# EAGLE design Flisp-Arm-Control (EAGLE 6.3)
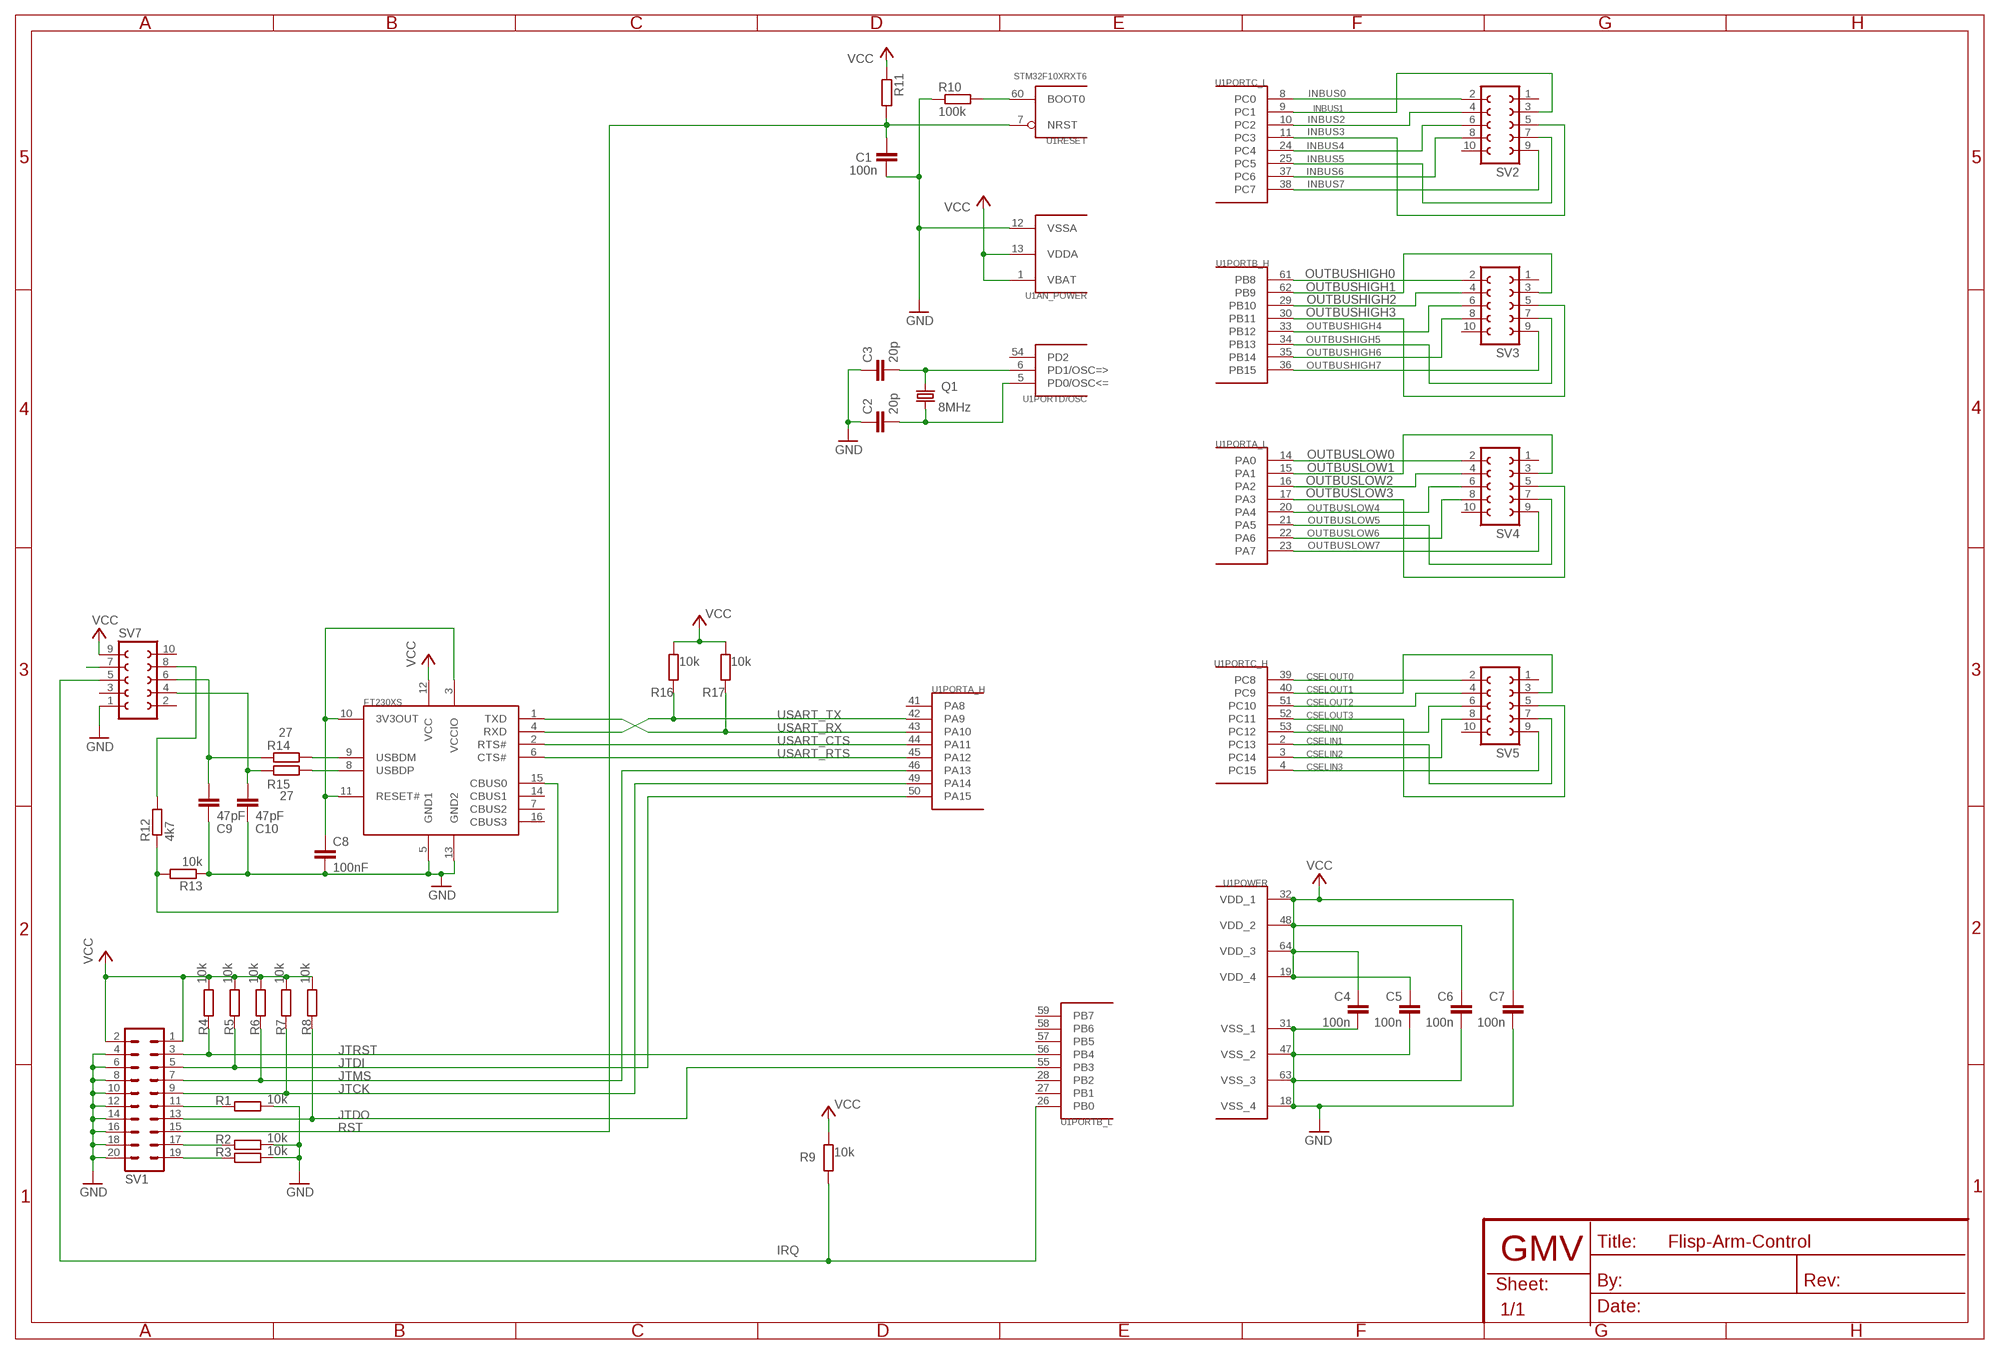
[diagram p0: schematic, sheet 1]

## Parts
C1  100n  C-EUC0603  [C0603]
C2  20p  C-EUC0603  [C0603]
C3  20p  C-EUC0603  [C0603]
C4  100n  C-EUC0603  [C0603]
C5  100n  C-EUC0603  [C0603]
C6  100n  C-EUC0603  [C0603]
C7  100n  C-EUC0603  [C0603]
C8  100nF  C-EUC0603  [C0603]
C9  47pF  C-EUC0603  [C0603]
C10  47pF  C-EUC0603  [C0603]
Q1  8MHz  CRYSTALSM49  [SM49]
R1  10k  R-EU_R0603  [R0603]
R2  10k  R-EU_R0603  [R0603]
R3  10k  R-EU_R0603  [R0603]
R4  10k  R-EU_R0603  [R0603]
R5  10k  R-EU_R0603  [R0603]
R6  10k  R-EU_R0603  [R0603]
R7  10k  R-EU_R0603  [R0603]
R8  10k  R-EU_R0603  [R0603]
R9  10k  R-EU_R0603  [R0603]
R10  100k  R-EU_R0603  [R0603]
R11  R-EU_R0603  [R0603]
R12  4k7  R-EU_R0603  [R0603]
R13  10k  R-EU_R0603  [R0603]
R14  27  R-EU_R0603  [R0603]
R15  27  R-EU_R0603  [R0603]
R16  10k  R-EU_R0603  [R0603]
R17  10k  R-EU_R0603  [R0603]
SV1  ML20  [ML20]
SV2  FE05-2  [FE05-2]
SV3  FE05-2  [FE05-2]
SV4  FE05-2  [FE05-2]
SV5  FE05-2  [FE05-2]
SV7  FE05-2  [FE05-2]
U1  STM32F10XRXT6  [TQFP64]
U2  FT230XS  [SSOP16-FTDI]

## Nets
CSELIN0: SV5.6 U1.53(PORTC_H:PC12)
CSELIN1: SV5.7 U1.2(PORTC_H:PC13)
CSELIN2: SV5.8 U1.3(PORTC_H:PC14)
CSELIN3: SV5.9 U1.4(PORTC_H:PC15)
CSELOUT0: SV5.2 U1.39(PORTC_H:PC8)
CSELOUT1: SV5.3 U1.40(PORTC_H:PC9)
CSELOUT2: SV5.4 U1.51(PORTC_H:PC10)
CSELOUT3: SV5.5 U1.52(PORTC_H:PC11)
GND: C1.1 C2.1 C3.1 C4.2 C5.2 C6.2 C7.2 C8.2 C9.2 C10.2 R1.2 R2.2 R3.2 R10.1 R13.1 SV1.4 SV1.6 SV1.8 SV1.10 SV1.12 SV1.14 SV1.16 SV1.18 SV1.20 SV7.1 U1.12(AN_POWER:VSSA) U1.18(POWER:VSS_4) U1.31(POWER:VSS_1) U1.47(POWER:VSS_2) U1.63(POWER:VSS_3) U2.5(GND1) U2.13(GND2)
INBUS0: SV2.2 U1.8(PORTC_L:PC0)
INBUS1: SV2.3 U1.9(PORTC_L:PC1)
INBUS2: SV2.4 U1.10(PORTC_L:PC2)
INBUS3: SV2.5 U1.11(PORTC_L:PC3)
INBUS4: SV2.6 U1.24(PORTC_L:PC4)
INBUS5: SV2.7 U1.25(PORTC_L:PC5)
INBUS6: SV2.8 U1.37(PORTC_L:PC6)
INBUS7: SV2.9 U1.38(PORTC_L:PC7)
IRQ: R9.1 SV7.5 U1.26(PORTB_L:PB0)
JTCK: R7.1 SV1.9 U1.49(PORTA_H:PA14)
JTDI: R5.1 SV1.5 U1.50(PORTA_H:PA15)
JTDO: R8.1 SV1.13 U1.55(PORTB_L:PB3)
JTMS: R6.1 SV1.7 U1.46(PORTA_H:PA13)
JTRST: R4.1 SV1.3 U1.56(PORTB_L:PB4)
N$2: R10.2 U1.60(RESET:BOOT0)
N$3: R12.2 SV7.8
N$4: SV7.7
N$319: R14.2 U2.9(USBDM)
N$321: R15.2 U2.8(USBDP)
N$322: C3.2 Q1.2 U1.6(PORTD/OSC:PD1/OSC=>)
N$323: C2.2 Q1.1 U1.5(PORTD/OSC:PD0/OSC<=)
N$325: R3.1 SV1.19
N$334: R2.1 SV1.17
N$336: R1.1 SV1.11
N$337: C8.1 U2.3(VCCIO) U2.10(3V3OUT) U2.11(RESET#)
N$352: R12.1 R13.2 U2.15(CBUS0)
N$354: C9.1 R14.1 SV7.6
N$355: C10.1 R15.1 SV7.4
OUTBUSHIGH0: SV3.2 U1.61(PORTB_H:PB8)
OUTBUSHIGH1: SV3.3 U1.62(PORTB_H:PB9)
OUTBUSHIGH2: SV3.4 U1.29(PORTB_H:PB10)
OUTBUSHIGH3: SV3.5 U1.30(PORTB_H:PB11)
OUTBUSHIGH4: SV3.6 U1.33(PORTB_H:PB12)
OUTBUSHIGH5: SV3.7 U1.34(PORTB_H:PB13)
OUTBUSHIGH6: SV3.8 U1.35(PORTB_H:PB14)
OUTBUSHIGH7: SV3.9 U1.36(PORTB_H:PB15)
OUTBUSLOW0: SV4.2 U1.14(PORTA_L:PA0)
OUTBUSLOW1: SV4.3 U1.15(PORTA_L:PA1)
OUTBUSLOW2: SV4.4 U1.16(PORTA_L:PA2)
OUTBUSLOW3: SV4.5 U1.17(PORTA_L:PA3)
OUTBUSLOW4: SV4.6 U1.20(PORTA_L:PA4)
OUTBUSLOW5: SV4.7 U1.21(PORTA_L:PA5)
OUTBUSLOW6: SV4.8 U1.22(PORTA_L:PA6)
OUTBUSLOW7: SV4.9 U1.23(PORTA_L:PA7)
RST: C1.2 R11.2 SV1.15 U1.7(RESET:NRST)
USART_CTS: U1.44(PORTA_H:PA11) U2.2(RTS#)
USART_RTS: U1.45(PORTA_H:PA12) U2.6(CTS#)
USART_RX: R17.1 U1.43(PORTA_H:PA10) U2.1(TXD)
USART_TX: R16.1 U1.42(PORTA_H:PA9) U2.4(RXD)
VCC: C4.1 C5.1 C6.1 C7.1 R4.2 R5.2 R6.2 R7.2 R8.2 R9.2 R11.1 R16.2 R17.2 SV1.1 SV1.2 SV7.9 U1.1(AN_POWER:VBAT) U1.13(AN_POWER:VDDA) U1.19(POWER:VDD_4) U1.32(POWER:VDD_1) U1.48(POWER:VDD_2) U1.64(POWER:VDD_3) U2.12(VCC)
Unconnected: SV2.1 SV2.10 SV3.1 SV3.10 SV4.1 SV4.10 SV5.1 SV5.10 SV7.2 SV7.3 SV7.10 U1.27(PORTB_L:PB1) U1.28(PORTB_L:PB2) U1.41(PORTA_H:PA8) U1.54(PORTD/OSC:PD2) U1.57(PORTB_L:PB5) U1.58(PORTB_L:PB6) U1.59(PORTB_L:PB7) U2.7(CBUS2) U2.14(CBUS1) U2.16(CBUS3)

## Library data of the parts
C1-C10 = rcl:C-EU: CAPACITOR, European symbol
Q1 = crystal:CRYSTAL: CRYSTAL; OC_FARNELL: unknown; OC_NEWARK: unknown
R1-R17 = rcl:R-EU_: RESISTOR, European symbol
SV1 = con-harting-ml:ML20: HARTING; OC_FARNELL: unknown; OC_NEWARK: unknown
SV2-SV5 SV7 = con-lsta:FE05-2: FEMALE HEADER; OC_FARNELL: unknown; OC_NEWARK: unknown
U1 = stm32:STM32F10XRXT6: STM32F101/103 64pin LQFP
U2 = 0misc:FT230X

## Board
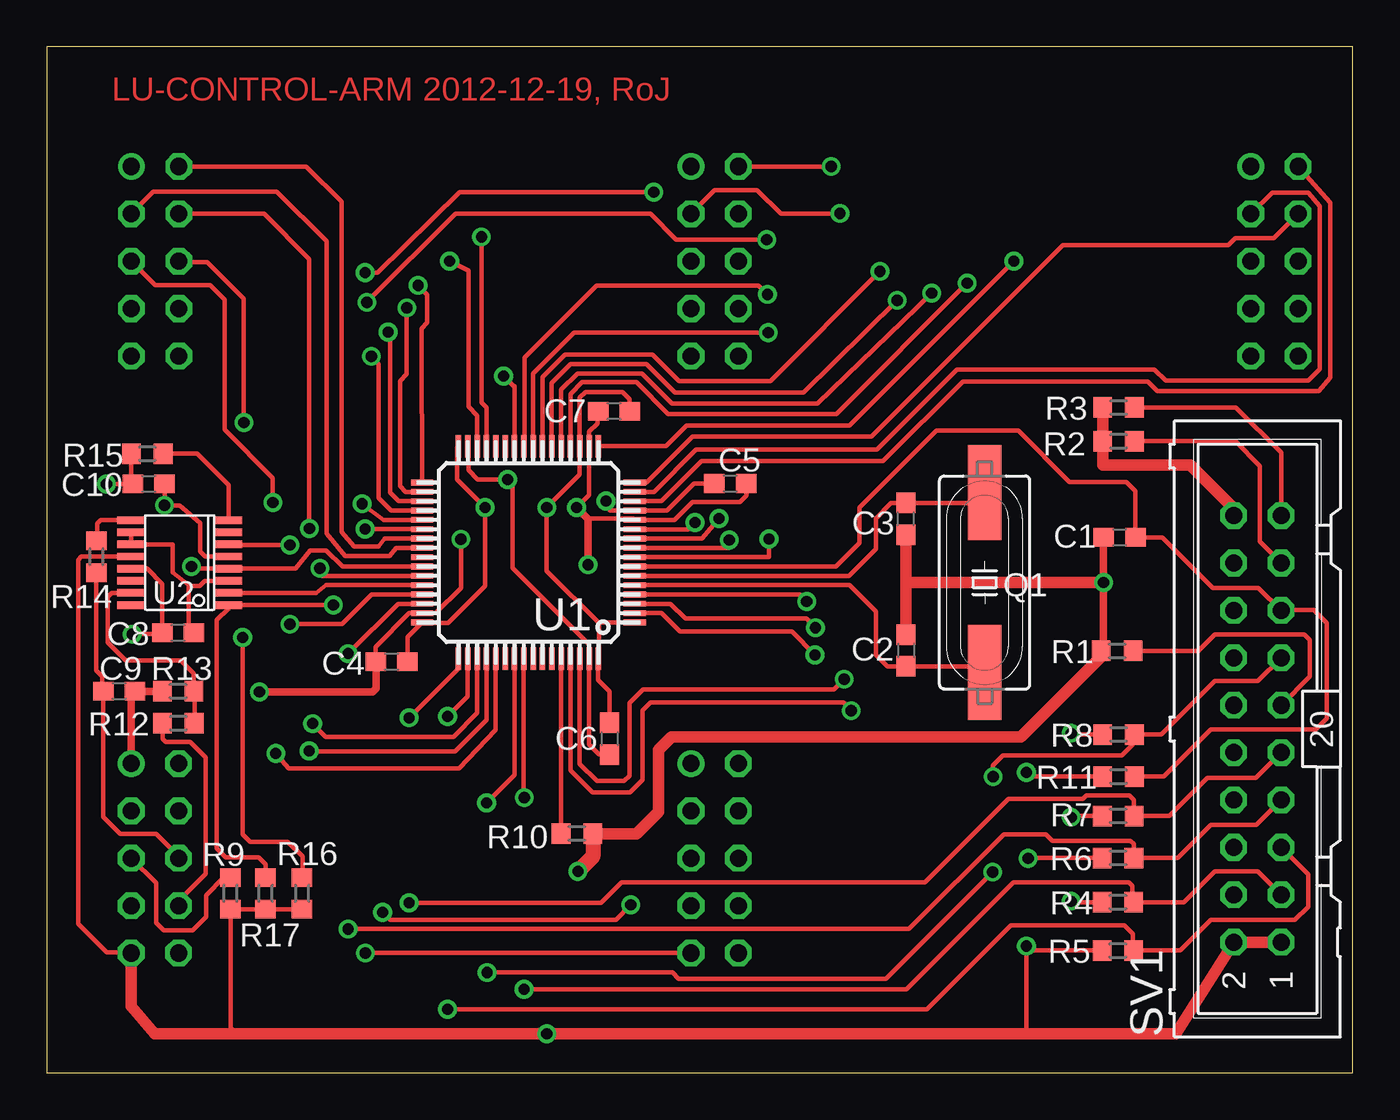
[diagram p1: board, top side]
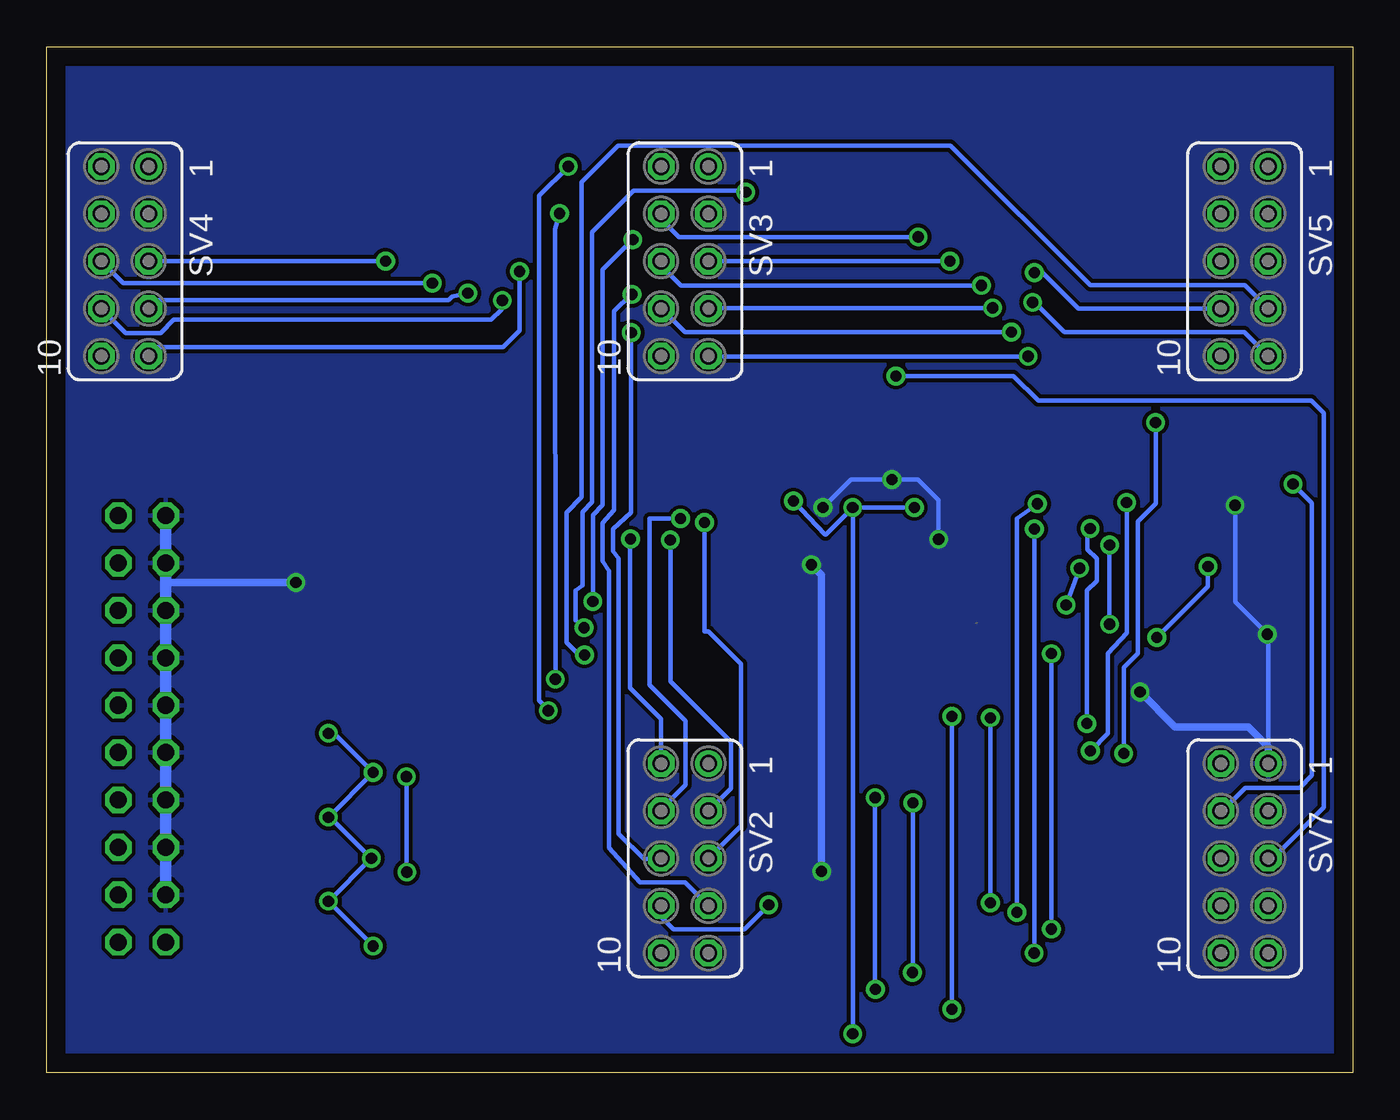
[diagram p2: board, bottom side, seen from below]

Size 70 x 55 mm. Coordinates in mm from the lower left corner, seen from the top.
Outline: 0,0 70,0 70,55 0,55 0,0
Copper layers (1*16): Top 0.035mm / dielectric 1.5mm / Bottom 0.035mm
Design rules "default *": minimum track width 10mil, minimum drill 12mil, track to track 8mil, track to pad 8mil, pad to pad 8mil, via to via 8mil, smd to smd 0mil, copper to edge 40mil, drill to drill 8mil, minimum pad ring 10mil, minimum via ring 8mil, stop-mask expansion 4mil, vias tented up to drill 0mil, thermal gap 10mil

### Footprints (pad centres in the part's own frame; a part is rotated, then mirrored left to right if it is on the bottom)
C0603 = smd 1.1 x 1: 1 -0.85,0; 2 0.85,0
SM49 = smd 5.08 x 1.778: 1 -4.826,0; 2 4.826,0
R0603 = smd 1 x 1.1: 1 -0.85,0; 2 0.85,0
ML20 = drill 0.914 octagon: 1 -11.43,-1.27; 2 -11.43,1.27; 3 -8.89,-1.27; 4 -8.89,1.27; 5 -6.35,-1.27; 6 -6.35,1.27; 7 -3.81,-1.27; 8 -3.81,1.27; 9 -1.27,-1.27; 10 -1.27,1.27; 11 1.27,-1.27; 12 1.27,1.27; 13 3.81,-1.27; 14 3.81,1.27; 15 6.35,-1.27; 16 6.35,1.27; 17 8.89,-1.27; 18 8.89,1.27; 19 11.43,-1.27; 20 11.43,1.27
FE05-2 = drill 0.914: 1 -5.08,1.27 | drill 0.914 octagon: 2 -5.08,-1.27; 3 -2.54,1.27; 4 -2.54,-1.27; 5 0,1.27; 6 0,-1.27; 7 2.54,1.27; 8 2.54,-1.27; 9 5.08,1.27; 10 5.08,-1.27
TQFP64 = smd 1.2 x 0.3: 1 -5.7,3.75; 2 -5.7,3.25; 3 -5.7,2.75; 4 -5.7,2.25; 5 -5.7,1.75; 6 -5.7,1.25; 7 -5.7,0.75; 8 -5.7,0.25; 9 -5.7,-0.25; 10 -5.7,-0.75; 11 -5.7,-1.25; 12 -5.7,-1.75; 13 -5.7,-2.25; 14 -5.7,-2.75; 15 -5.7,-3.25; 16 -5.7,-3.75; 33 5.7,-3.75; 34 5.7,-3.25; 35 5.7,-2.75; 36 5.7,-2.25; 37 5.7,-1.75; 38 5.7,-1.25; 39 5.7,-0.75; 40 5.7,-0.25; 41 5.7,0.25; 42 5.7,0.75; 43 5.7,1.25; 44 5.7,1.75; 45 5.7,2.25; 46 5.7,2.75; 47 5.7,3.25; 48 5.7,3.75 | smd 0.3 x 1.2: 17 -3.75,-5.7; 18 -3.25,-5.7; 19 -2.75,-5.7; 20 -2.25,-5.7; 21 -1.75,-5.7; 22 -1.25,-5.7; 23 -0.75,-5.7; 24 -0.25,-5.7; 25 0.25,-5.7; 26 0.75,-5.7; 27 1.25,-5.7; 28 1.75,-5.7; 29 2.25,-5.7; 30 2.75,-5.7; 31 3.25,-5.7; 32 3.75,-5.7; 49 3.75,5.7; 50 3.25,5.7; 51 2.75,5.7; 52 2.25,5.7; 53 1.75,5.7; 54 1.25,5.7; 55 0.75,5.7; 56 0.25,5.7; 57 -0.25,5.7; 58 -0.75,5.7; 59 -1.25,5.7; 60 -1.75,5.7; 61 -2.25,5.7; 62 -2.75,5.7; 63 -3.25,5.7; 64 -3.75,5.7
SSOP16-FTDI = smd 0.4 x 1.5: 1 -2.275,-2.609; 2 -1.625,-2.609; 3 -0.975,-2.609; 4 -0.325,-2.609; 5 0.325,-2.609; 6 0.975,-2.609; 7 1.625,-2.609; 8 2.275,-2.609; 9 2.275,2.609; 10 1.625,2.609; 11 0.975,2.609; 12 0.325,2.609; 13 -0.325,2.609; 14 -0.975,2.609; 15 -1.625,2.609; 16 -2.275,2.609

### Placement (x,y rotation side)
C1  57.5,28.7 0 top
C2  46.05,22.64 270 top
C3  46.05,29.7 90 top
C4  18.49,22.03 180 top
C5  36.63,31.58 0 top
C6  30.17,17.91 270 top
C7  30.4,35.46 180 top
C8  7.05,23.58 180 top
C9  3.89,20.46 0 top
C10  5.47,31.57 0 top
Q1  50.27,26.28 90 top
R1  57.37,22.62 180 top
R2  57.44,33.85 180 top
R3  57.44,35.66 180 top
R4  57.41,9.15 180 top
R5  57.4,6.55 180 top
R6  57.41,11.52 180 top
R7  57.43,13.77 180 top
R8  57.44,18.14 180 top
R9  9.85,9.62 270 top
R10  28.42,12.83 180 top
R11  57.44,15.88 0 top
R12  7.06,18.74 180 top
R13  7.05,20.45 0 top
R14  2.67,27.66 90 top
R15  5.39,33.18 0 top
R16  13.69,9.62 270 top
R17  11.73,9.62 270 top
SV1  64.89,18.43 90 top
SV2  35.8,11.5 270 bottom
SV3  35.8,43.5 270 bottom
SV4  65.8,43.5 270 bottom
SV5  5.81,43.5 270 bottom
SV7  5.8,11.5 270 bottom
U1  25.82,27.89 180 top
U2  7.13,27.35 90 top

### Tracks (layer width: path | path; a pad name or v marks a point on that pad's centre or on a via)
CSELIN0  (via drill 0.6)
  Top 0.254: U1.53 24.07,18.38 22.11,16.32 12.98,16.32 v12.28,17.12 | v10.57,34.85 10.57,41.49 8.6,43.46 7.12,43.46 SV5.6
  Bottom 0.254: v12.28,17.12 12.28,21.72 11.53,22.47 11.53,29.56 10.57,30.52 v10.57,34.85
CSELIN1  (via drill 0.6)
  Top 0.254: U1.2 32.94,24.64 33.93,23.65 39.93,23.65 v41.18,22.4
  Bottom 0.254: v41.18,22.4 41.46,22.4 42.14,23.08 42.14,30.04 41.33,30.85 41.33,47.75 39.39,49.69 21.56,49.69 14.08,42.21 5.79,42.21 SV5.7
CSELIN2  (via drill 0.6)
  Top 0.254: U1.3 33.43,25.14 34.23,24.34 40.72,24.34 v41.2,23.86 | v32.54,47.2 22.12,47.2 17.74,42.9 v17.08,42.9 v17.07,42.89
  Bottom 0.254: v41.2,23.86 41.2,23.89 41.66,24.25 41.66,25.86 41.29,26.13 41.29,30.07 40.77,30.59 40.77,45.05 38.55,47.27 32.61,47.27 v32.54,47.2 | v17.07,42.89 16.65,42.89 14.71,40.95 SV5.8
CSELIN3  (via drill 0.6)
  Top 0.254: U1.4 40.36,25.64 v40.73,25.27 | v38.59,44.66 33.74,44.66 32.35,46.05 21.91,46.05 v17.16,41.3
  Bottom 0.254: v40.73,25.27 40.73,29.91 40.2,30.44 40.2,43.05 v38.59,44.66 | v17.16,41.3 17.07,41.3 15.46,39.69 5.81,39.69 SV5.9
CSELOUT0
  Top 0.254: U1.39 18.1,28.64 17.78,28.22 16.48,28.22 15.8,29 15.8,46.69 13.91,48.58 SV5.2
CSELOUT1
  Top 0.254: U1.40 18.72,28.14 18.38,27.7 16,27.7 15,28.9 15,44.57 12.33,47.24 5.72,47.24 4.54,46.06 SV5.3
CSELOUT2  (via drill 0.6)
  Top 0.254: U1.51 23.07,19.28 21.8,18.01 14.96,18.01 v14.25,18.72 | v14.08,29.18 14.08,43.62 11.66,46.04 SV5.4
  Bottom 0.254: v14.25,18.72 14.25,25.85 13.73,26.37 13.73,27.56 14.23,28.06 14.23,29.03 v14.08,29.18
CSELOUT3  (via drill 0.6)
  Top 0.254: U1.52 23.57,18.91 21.9,17.24 v14.07,17.24 v14.06,17.25 | v12.12,30.56 12.12,31.89 9.53,34.48 9.53,41.44 8.75,42.22 5.82,42.22 SV5.5
  Bottom 0.254: v14.06,17.25 v14.05,17.25 13.12,18.18 13.12,22.47 12.12,23.57 v12.12,30.56
GND  (via drill 0.6)
  Top 0.254: C6.2 29.6,17.06 29.06,17.6 U1.63 29.07,22.95 24.97,27.05 24.97,31.53 v24.7,31.8 23.1,31.8 22.6,32.3 22.6,33.56 U1.31 | C4.2 17.62,22.05 17.62,22.83 19.43,24.64 U1.47 20.84,24.64 22.2,26 v22.2,28.6 | C7.2 29.51,35.42 29.51,34.81 29.07,34.37 U1.18 29.07,30.97 v28.4,30.3 29,29.7 31.46,29.7 U1.12 33.64,29.64 34.6,30.6 37.15,30.6 37.5,30.95 37.5,31.56 C5.2 | U2.13 5.38,27.02 6.2,26.2 C8.2 6.13,23.51 v4.59,23.51 | 4.53,20.25 C9.2 R13.1 | C10.2 v6.32,30.43 v6.31,30.42 6.33,30.4 7.12,30.4 8.24,29.48 8.24,27.94 8.51,27.68 U2.5
  Top 0.406: C1.1 56.61,28.74 56.58,28.74 56.64,28.68 v56.64,26.28 56.64,22.74 R1.2 | v29.01,27.23 29.01,29.69 v28.4,30.3 | v11.4,20.42 17.46,20.42 17.65,20.61 C4.2 | R13.1 4.53,20.45 SV7.1
  Top 0.61: C2.1 C3.1 46.05,26.28 v56.64,26.28 | R3.2 R2.2 56.59,32.57 61.3,32.57 63.62,30.25 SV1.20 | 56.64,22.74 56.64,22.43 52.22,18.01 33.48,18.01 32.79,17.32 32.79,14 31.61,12.82 R10.1
  Top 0.813: R10.1 29.27,11.6 v28.47,10.8
  Bottom 0.254: v22.2,28.6 22.2,30.7 23.3,31.8 v24.7,31.8 26.9,31.8 v28.4,30.3 | v6.31,30.42 6.31,25.23 v4.59,23.51 4.53,23.45 SV7.1
  Bottom 0.406: v56.64,26.28 63.62,26.28 | v28.47,10.8 28.47,26.69 v29.01,27.23 | SV7.1 4.53,17.48 5.6,18.55 9.53,18.55 v11.4,20.42
  Bottom 0.61: SV1.4 SV1.6 SV1.8 SV1.10 SV1.12 SV1.14 SV1.16 63.62,26.28 SV1.18 SV1.20
  pour Bottom: 0,55 70,55 70,0 0,0
INBUS0  (via drill 0.6)
  Top 0.254: U1.8 38.71,27.65 v38.71,28.61
  Bottom 0.254: SV2.2 37.07,18.96 38.74,20.63 38.74,28.58 v38.71,28.61
INBUS1  (via drill 0.6)
  Top 0.254: U1.9 36.38,28.14 36.58,28.13 v36.58,28.56
  Bottom 0.254: v36.58,28.56 36.58,20.99 33.32,17.73 33.32,15.25 SV2.3
INBUS2  (via drill 0.6)
  Top 0.254: v36.03,29.71 35.12,28.64 U1.10
  Bottom 0.254: v36.03,29.71 37.69,29.71 37.69,20.79 35.77,18.87 35.77,15.42 37.07,14.12 SV2.4
INBUS3  (via drill 0.6)
  Top 0.254: U1.11 34.38,29.13 v34.75,29.5
  Bottom 0.254: v34.75,29.5 34.74,23.66 34.53,23.66 32.78,21.91 32.78,13.25 SV2.5
INBUS4  (via drill 0.6)
  Top 0.254: 26.1,33.62 U1.24 26.07,37.48 28.27,39.68 v38.66,39.68 v38.67,39.67
  Bottom 0.254: v38.67,39.67 38.67,30.03 39.65,29.15 39.65,27.97 39.36,27.58 39.36,12.82 38,11.46 37.11,11.46 SV2.6
INBUS5  (via drill 0.6)
  Top 0.254: U1.25 25.6,33.62 25.6,38.34 29.46,42.2 38.15,42.2 v38.63,41.72
  Bottom 0.254: v38.63,41.72 38.69,41.72 39.59,40.82 39.59,30.17 40.2,29.46 40.2,27.44 39.86,26.9 39.86,12.07 38.21,10.22 35.79,10.22 SV2.7
INBUS6  (via drill 0.6)
  Top 0.254: U1.37 18.06,29.64 v16.9,30.5 | v18,8.6 18.4,8.2 30.5,8.2 v31.3,9
  Bottom 0.254: v16.9,30.5 18,29.7 v18,8.6 | v31.3,9 32.6,7.7 36.4,7.7 37.07,8.37 SV2.8
INBUS7  (via drill 0.6)
  Top 0.254: U1.38 v17.06,29.14 | v17.08,6.42 SV2.9
  Bottom 0.254: v17.06,29.14 17.07,20.82 v17.07,6.43 v17.08,6.42
IRQ  (via drill 0.6)
  Top 0.254: U1.26 25.07,36.81 25.03,36.81 v24.49,37.35 | R9.1 9.49,10.47 8.54,9.52 8.54,8.36 7.82,7.64 6.26,7.64 5.86,8.04 5.86,10.17 SV7.5
  Bottom 0.254: v24.49,37.35 18.18,37.35 16.86,36.03 2.22,36.03 1.56,35.37 1.56,14.24 4.3,11.5 SV7.5
JTCK  (via drill 0.6)
  Top 0.254: SV1.9 64.79,15.8 62.2,15.8 60.17,13.77 R7.1 58.26,13.79 58.26,14.62 58.02,14.86 55.72,14.86 55.53,14.67 51.53,14.67 47.08,10.22 33.72,10.22 30.81,10.21 29.7,9.1 v19.43,9.11 | U1.49 22.07,21.67 v19.43,19.03
  Bottom 0.254: v19.43,19.03 v19.43,9.11
JTDI  (via drill 0.6)
  Top 0.254: SV1.5 67.6,10.64 67.6,8.9 66.9,8.2 62.4,8.2 60.76,6.55 R5.1 58.22,6.59 58.22,7.45 57.76,7.91 51.68,7.91 47.18,3.41 v21.49,3.41 | U1.50 22.57,20.18 v21.49,19.1
  Bottom 0.254: v21.49,19.1 v21.49,3.41
JTDO  (via drill 0.6)
  Top 0.254: SV1.13 64.91,21 62.6,21 59.74,18.14 R8.1 58.22,18.21 58.22,17.6 57.63,17.01 51.24,17.01 50.72,16.49 v50.72,15.88 | U1.55 25.07,15.96 v23.58,14.47 | v23.61,5.38 33.53,5.38 33.86,5.05 44.99,5.05 v50.7,10.76
  Bottom 0.254: v23.58,14.47 23.58,5.41 v23.61,5.38 | v50.7,10.76 50.7,15.86 v50.72,15.88
JTMS  (via drill 0.6)
  Top 0.254: SV1.7 64.83,13.3 62.4,13.3 60.62,11.52 R6.1 58.25,12.27 58.08,12.44 53.9,12.44 53.56,12.78 51.29,12.78 46.22,7.71 v16.15,7.71 | U1.46 18.83,25.14 v16.16,22.47
  Bottom 0.254: v16.16,22.47 v16.16,7.72 v16.15,7.71
JTRST  (via drill 0.6)
  Top 0.254: SV1.3 64.9,10.8 62.6,10.8 60.95,9.15 R4.1 58.19,9.21 58.19,10.01 57.99,10.21 51.8,10.21 46.07,4.48 v25.58,4.48 | U1.56 25.57,14.78 v25.6,14.75
  Bottom 0.254: v25.6,14.75 25.6,4.5 v25.58,4.48
N$2
  Top 0.254: U1.60 R10.2
N$3
  Top 0.254: SV7.8 7.07,9.22 8.51,10.66 8.51,16.91 7.69,17.73 6.39,17.73 6.21,17.91 R12.2
N$319
  Top 0.254: U2.9 2.9,29.62 2.7,29.43 2.7,28.61 R14.2
N$321
  Top 0.254: R15.2 8.08,33.18 9.75,31.51 9.75,29.64 U2.8
N$322
  Top 0.254: U1.6 43,26.64 44.44,28.08 44.44,29.72 45.25,30.53 46.03,30.53 C3.2 49.71,30.55 | Q1.2 49.83,30.67 49.71,30.55 | 49.71,30.55 49.5,30.34
N$323
  Top 0.254: U1.5 43.02,26.14 44.44,24.72 44.44,22.41 45.07,21.78 C2.2 49.93,21.79 Q1.1
N$325
  Top 0.254: R3.1 63.74,35.66 66.16,33.24 SV1.19
N$334
  Top 0.254: R2.1 63.69,33.85 65.01,32.53 65.01,28.47 SV1.17
N$336
  Top 0.254: R1.1 61.72,22.62 62.6,23.5 67.4,23.5 67.7,23.2 67.7,21.25 SV1.11
N$337
  Top 0.254: U2.10 U2.11 4.54,28.31 6.76,28.31 6.76,26.83 7.61,26.16 7.6,26.18 | C8.1 7.6,23.88 7.6,26.18 | U2.3 8.47,26.38 8.2,26.1 7.67,26.1 7.6,26.18
N$352
  Top 0.254: R12.1 7.91,18.8 7.92,18.81 7.92,20.43 R13.2 7.88,20.47 7.88,21.41 7.19,22.1 4.23,22.1 3.26,23.07 3.26,25.5 3.48,25.73 U2.15
N$354
  Top 0.254: SV7.6 7.07,11.59 5.86,12.8 3.95,12.8 3.03,13.72 C9.1 2.99,20.51 2.99,21.24 2.67,21.56 R14.1
N$355  (via drill 0.6)
  Top 0.254: v3.21,31.56 C10.1 4.54,31.64 R15.1
  Bottom 0.254: SV7.4 7.01,14.04 5.77,15.28 2.85,15.28 2.2,15.93 2.2,30.55 v3.21,31.56
OUTBUSHIGH0  (via drill 0.6)
  Top 0.254: U1.61 28.07,16.2 29.25,15.02 31.26,15.02 31.94,15.7 31.94,19.43 32.35,19.84 42.69,19.84 v43.12,19.41 | v42.04,48.58 SV3.2
  Bottom 0.254: v43.12,19.41 43.12,19.47 43.61,19.96 43.61,47.01 v42.04,48.58
OUTBUSHIGH1  (via drill 0.6)
  Top 0.254: U1.62 28.57,16.56 29.49,15.64 30.95,15.64 31.23,15.92 31.23,19.82 31.96,20.55 42.19,20.55 v42.74,21.1 | v42.51,46.06 39.34,46.04 38.08,47.3 35.79,47.3 SV3.3
  Bottom 0.254: v42.74,21.1 42.76,45.21 v42.51,46.06
OUTBUSHIGH2  (via drill 0.6)
  Top 0.254: U1.29 23.57,35.65 23.3,35.92 v23.3,44.8
  Bottom 0.254: SV3.4 37.07,45.77 36.1,44.8 v23.3,44.8
OUTBUSHIGH3  (via drill 0.6)
  Top 0.254: U1.30 23.07,35.24 22.6,35.71 22.6,43 v21.59,43.51
  Bottom 0.254: v21.59,43.51 SV3.5
OUTBUSHIGH4  (via drill 0.6)
  Top 0.254: v19.9,42.2 20.4,41.7 20.4,40.2 20.1,39.9 20.1,39 U1.33
  Bottom 0.254: SV3.6 37.17,43.4 37.2,43.4 36,42.2 v19.9,42.2
OUTBUSHIGH5  (via drill 0.6)
  Top 0.254: U1.34 19.24,31.14 18.93,31.45 18.93,37.08 19.3,37.45 v19.3,41
  Bottom 0.254: SV3.7 34.49,41 21.1,41 21,41 v19.3,41
OUTBUSHIGH6  (via drill 0.6)
  Top 0.254: U1.35 18.86,30.64 18.4,31.1 18.4,39.6 v18.3,39.7
  Bottom 0.254: SV3.8 37.1,40.99 37.1,41 35.8,39.7 20.8,39.7 20.5,39.7 v18.3,39.7
OUTBUSHIGH7  (via drill 0.6)
  Top 0.254: U1.36 18.46,30.14 17.8,30.8 17.8,38 v17.4,38.4
  Bottom 0.254: SV3.9 34.51,38.4 v17.4,38.4
OUTBUSLOW0
  Top 0.254: U1.14 32.94,30.64 35.1,32.8 44.83,32.8 49.09,37.06 59,37.06 59.52,36.54 68.17,36.54 68.8,37.27 68.8,46.65 SV4.2
OUTBUSLOW1
  Top 0.254: U1.15 32.54,31.14 34.8,33.4 44.5,33.4 48.79,37.69 59.37,37.69 59.97,37.09 67.61,37.09 68.24,37.72 68.24,46.46 67.62,47.18 65.67,47.18 SV4.3
OUTBUSLOW2
  Top 0.254: U1.16 32.14,31.64 34.6,34.1 44.2,34.1 54.47,44.37 63.33,44.37 63.69,44.73 65.76,44.73 SV4.4
OUTBUSLOW3  (via drill 0.6)
  Top 0.254: U1.17 33.19,33.59 34.29,34.69 43.03,34.69 v51.84,43.5
  Bottom 0.254: v51.84,43.5 SV4.5
OUTBUSLOW4  (via drill 0.6)
  Top 0.254: U1.20 28.07,36.39 28.69,37.01 31.62,37.01 33.31,35.32 36.77,35.32 | 36.77,35.32 36.78,35.31 | 36.77,35.32 42.33,35.32 v49.33,42.32
  Bottom 0.254: v49.33,42.32 65.89,42.32 SV4.6
OUTBUSLOW5  (via drill 0.6)
  Top 0.254: U1.21 27.57,36.61 28.44,37.48 31.9,37.48 33.52,35.86 41.3,35.86 v47.43,41.79
  Bottom 0.254: v47.43,41.79 48.28,41.59 48.46,41.41 64.08,41.41 SV4.7
OUTBUSLOW6  (via drill 0.6)
  Top 0.254: U1.22 27.07,36.97 28.08,37.98 32.15,37.98 33.67,36.46 36.73,36.46 36.74,36.47 40.55,36.47 v45.58,41.4
  Bottom 0.254: v45.58,41.4 45.63,40.9 46.17,40.36 63.18,40.36 63.88,39.66 65.77,39.66 SV4.8
OUTBUSLOW7  (via drill 0.6)
  Top 0.254: U1.23 26.57,37.29 27.78,38.5 32.46,38.5 33.88,37.08 38.78,37.08 v44.66,42.96
  Bottom 0.254: v44.66,42.96 44.66,39.79 45.54,38.91 64.04,38.91 SV4.9
RST
  Top 0.254: U1.7 42.31,27.14 43.56,28.39 43.56,30.3 47.68,34.42 52.07,34.42 54.82,31.67 57.87,31.67 58.35,31.19 C1.2 | 58.28,28.77 C1.2 | R11.2 59.88,15.88 62.4,18.4 68,18.4 68.6,19 68.6,24.1 67.9,24.8 66.17,24.8 SV1.15 64.94,26 62.5,26 59.8,28.7 C1.2
USART_CTS
  Top 0.254: U1.44 14.97,26.15 14.45,25.73 U2.2
USART_RTS  (via drill 0.6)
  Top 0.254: U2.6 9.77,28.29 v13.04,28.29 | v13.04,24.05 14.8,24.05 14.78,24.05 15.84,24.05 17.42,25.64 U1.45
  Bottom 0.254: v13.04,28.29 v13.04,24.05
USART_RX  (via drill 0.6)
  Top 0.254: U2.1 | U2.1 v15.37,25.07 | v14.64,27.05 14.75,26.64 U1.43 | U2.1 9.74,24.89 9.11,24.26 9.11,12.03 9.59,11.55 11.35,11.55 11.73,11.17 R17.1
  Bottom 0.254: v15.37,25.07 15.34,25.1 v14.64,27.05
USART_TX  (via drill 0.6)
  Top 0.254: U1.42 15.85,27.14 14.99,28 14.11,28 13.35,27.04 9.75,27.04 U2.4 7.88,27.02 v7.76,27.14 | v10.51,23.33 10.51,12.78 10.9,12.39 12.91,12.39 13.71,11.59 13.71,10.49 R16.1
  Bottom 0.254: v7.76,27.14 7.76,26.08 v10.51,23.33
VCC  (via drill 0.6)  (1 unrouted)
  Top 0.254: C6.1 30.17,20.45 29.56,21.06 U1.64 29.6,22.22 29.6,24.1 | C7.1 31.24,36.12 30.86,36.5 28.87,36.5 28.57,36.2 U1.19 28.57,32.07 v26.8,30.3 26.8,26.9 29.6,24.1 | R8.2 54.96,18.14 v54.9,18.2 | 52.5,2.1 v52.5,6.8 52.74,6.55 R5.2 | R4.2 54.95,9.15 v54.9,9.2 | R6.2 52.62,11.52 v52.6,11.5 | R7.2 54.97,13.77 v54.9,13.7 | R11.1 52.72,15.88 v52.5,16.1 | 20.2,24.1 21.5,24.1 23.5,26.1 v23.5,30.3 22,31.8 22,33.52 U1.32 | U1.1 29.64,24.14 29.6,24.1 | SV7.9 4.48,6.47 3.22,6.47 1.69,8 1.69,27.5 1.86,27.68 U2.12 | v29.98,30.64 30.18,30.14 U1.13 33.25,30.15 34.68,31.58 C5.1 | R16.2 R17.2 11.44,8.76 R9.2 9.85,2.42 10.17,2.1 | C4.1 19.34,23.36 U1.48
  Top 0.61: SV7.9 4.53,3.57 5.8,2.1 10.17,2.1 v26.8,2.1 52.5,2.1 60.51,2.1 SV1.2 SV1.1
  Bottom 0.254: v54.9,18.2 54.6,18.2 v52.5,16.1 v54.9,13.7 54.8,13.7 v52.6,11.5 v54.9,9.2 v52.5,6.8 | v26.8,30.3 v26.8,2.1 | v23.5,30.3 v26.8,30.3 | v29.98,30.64 28.3,28.86 28.24,28.86 v26.8,30.3

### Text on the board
Top: LU-CONTROL-ARM 2012-12-19, RoJ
